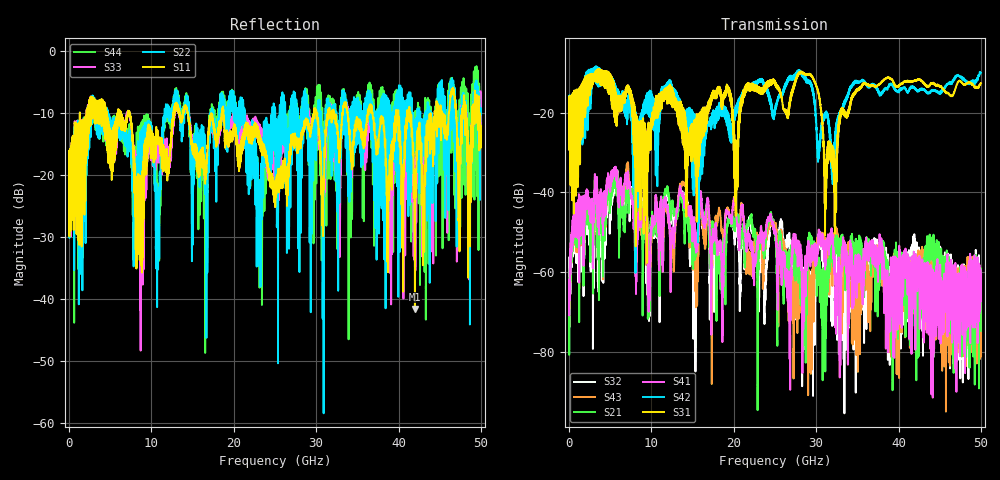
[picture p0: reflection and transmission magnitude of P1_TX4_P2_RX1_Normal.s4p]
!Keysight Technologies,N5225B,MY57041031,A.13.20.10
!Date: Friday, May 31, 2019 11:28:25
!Correction: S11(Full 4 Port(1,2,3,4))
!S12(Full 4 Port(1,2,3,4))
!S13(Full 4 Port(1,2,3,4))
!S14(Full 4 Port(1,2,3,4))
!S21(Full 4 Port(1,2,3,4))
!S22(Full 4 Port(1,2,3,4))
!S23(Full 4 Port(1,2,3,4))
!S24(Full 4 Port(1,2,3,4))
!S31(Full 4 Port(1,2,3,4))
!S32(Full 4 Port(1,2,3,4))
!S33(Full 4 Port(1,2,3,4))
!S34(Full 4 Port(1,2,3,4))
!S41(Full 4 Port(1,2,3,4))
!S42(Full 4 Port(1,2,3,4))
!S43(Full 4 Port(1,2,3,4))
!S44(Full 4 Port(1,2,3,4))
!S4P File: Measurements: <S11,S12,S13,S14>,
!<S21,S22,S23,S24>,
!<S31,S32,S33,S34>,
!<S41,S42,S43,S44>:
# Hz S  dB  R 50.0
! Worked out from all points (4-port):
!   5000 points, 10 MHz to 50 GHz, reference 50 ohm
!   strongest paths, dB at 10 MHz, 12.51 GHz, 25.01 GHz, 37.51 GHz, 50 GHz:
!     S31: -19.6, -17.9, -13.0, -13.1, -12.6
!     S42: -19.4, -14.1, -20.1, -14.5, -10.0
!     S41: -61.9, -49.4, -50.4, -57.4, -60.6
!     S21: -61.6, -42.9, -50.7, -66.0, -74.8
!     S43: -70.9, -52.7, -48.1, -56.7, -62.4
!     S32: -56.4, -44.8, -49.5, -55.0, -61.6
!   lowest |S11| = -41.6 dB at 41.99 GHz (marker M1), VSWR 1.02, Z = 50.8 - j0.109 ohm
!   |S11| at or under -10 dB: 7.334 GHz to 12.7 GHz (5.364 GHz wide, 53.5 % of centre); 14.41 GHz to 18.57 GHz (4.156 GHz wide, 25.2 % of centre); 18.74 GHz to 29.76 GHz (11.02 GHz wide, 45.4 % of centre)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
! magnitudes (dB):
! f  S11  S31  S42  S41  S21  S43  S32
! 10 MHz  -19.5  -19.6  -19.4  -61.9  -61.6  -70.9  -56.4
! 5.66 GHz  -12.8  -16.2  -16.5  -33.5  -35.8  -34.6  -36.3
! 20.25 GHz  -13.1  -33.6  -18.9  -45.1  -47.1  -44.6  -49.9
! 29.18 GHz  -13.0  -10.2  -12.5  -55.1  -51.3  -70.9  -62.0
! 32.24 GHz  -10.5  -36.0  -27.5  -60.1  -57.9  -51.0  -58.2
! 41.99 GHz  -41.6  -12.0  -13.8  -56.3  -64.4  -57.2  -51.7
! 50 GHz  -12.1  -12.6  -10.0  -60.6  -74.8  -62.4  -61.6
